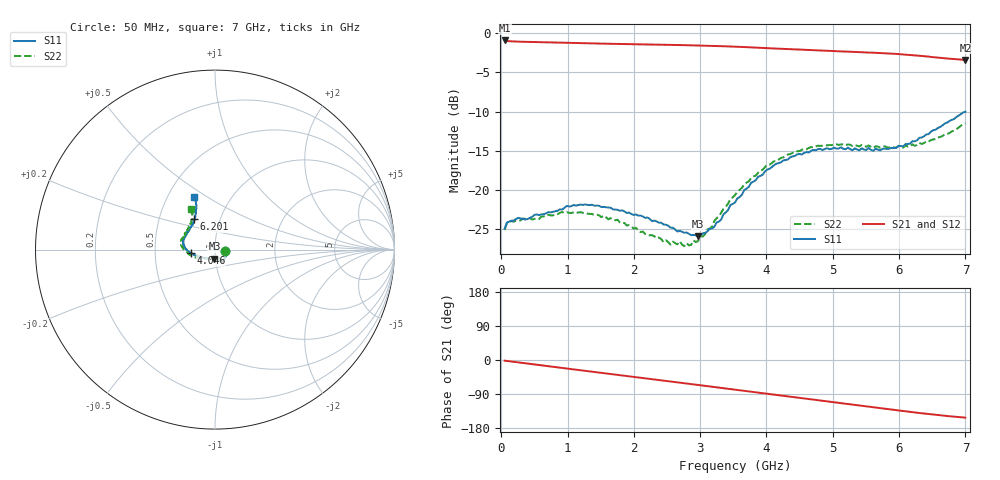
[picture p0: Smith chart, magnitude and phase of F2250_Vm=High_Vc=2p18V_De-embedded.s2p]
! Integrated Device Technology
! Corporate Headquarters
! 6024 Silver Creek Valley Road
! San Jose, CA 95138  USA
! Phone:  1-408-284-8200
! Toll Free:  1-800-223-1366
! Webpage:  http://www.idt.com/
! Timing and RF Division
! 515 Groton Road, Suite 102
! Westford, MA 01886-6024
! Device:  F2250
! Description: Voltage Variable RF Attenuator
! Frequency:  50.0 -  6000.00 MHz
! Package:  3x3 mm Thin QFN Plastic Package: 16 pin
! Ports:  2 RF, 3 DC
!  Pin  1  = GND
!  Pin  2  = NC
!  Pin  3  = RF1  = Port 1
!  Pin  4  = NC
!  Pin  5  = GND
!  Pin  6  = GND
!  Pin  7  = GND
!  Pin  8  = GND
!  Pin  9  = NC
!  Pin 10  = RF2  = Port 2
!  Pin 11  = NC
!  Pin 12  = GND
!  Pin 13  = GND
!  Pin 14  = VCNTRL
!  Pin 15  = VDD
!  Pin 16  = VMODE
! Vcntrl:  2.180 Volts
! Vmode:  +3.300 Volts
! Vdd:  +3.30  Volts
! Current:  1.316 mA
! Data:  The device was measured on a the F2250 evaluation board which has
!  individual transmission lines to the RF pins.  Data was collected
!  using a calibrated network analyzer.  The evaluation board was
!  de-embedded using a TRL calibration technique.
!  The reference plane is the edge of the package pin.
! Misc:  SN 10
!  Action Tracker AT0258
! Date Measured:  2014-11-26
! Date:  2015-10-15  MJV
! Note:
!  Integrated Device Technology supplies this data as a sample of measured
!  data at the package pin for this product.  Your particular data for this
!  product may vary.
!  Data was taken at 25 degrees C.
!  Integrated Device Technology reserves the right to change this data at anytime.
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# GHz S dB R 50
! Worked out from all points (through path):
!   201 points, 50 MHz to 7 GHz, reference 50 ohm
!   highest |S21| = -0.94 dB at 50 MHz (marker M1); lowest = -3.4 dB at 7 GHz (marker M2)
!   group delay of S21, straight-line fit = 61.1 ps
!   lowest |S11| = -25.9 dB at 2.969 GHz (marker M3), VSWR 1.11, Z = 49.4 - j5.01 ohm
!   |S11| at or under -10 dB: start of sweep to end of sweep
!   |S22| runs from -27.2 to -11.5 dB; largest |S21 - S12| = 0.0019
!   S11 on the Smith chart (normalised r, x): 50 MHz: 1.12, -0.02; 4.046 GHz: 0.76, -0.03; 6.201 GHz: 0.75, +0.26; 7 GHz: 0.68, +0.44
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0.05  -24.94 -9.8  -0.94 -1.8  -0.93 -1.8  -25.11 -10.2
0.1195  -24.03 -9.5  -1.03 -3.3  -1.03 -3.2  -24.01 -8.5
0.91875  -22.50 -47.8  -1.22 -21.0  -1.22 -21.1  -22.80 -49.6
1.2315  -21.90 -55.6  -1.29 -27.9  -1.29 -27.9  -22.91 -60.1
1.75275  -22.52 -62.5  -1.38 -39.1  -1.38 -39.1  -23.78 -67.0
2.37825  -24.18 -62.5  -1.47 -52.8  -1.47 -52.8  -26.07 -67.9
2.552  -24.80 -67.1  -1.49 -56.6  -1.49 -56.7  -26.97 -74.5
2.691  -25.22 -74.6  -1.52 -59.7  -1.52 -59.8  -26.54 -81.8
2.7605  -25.45 -76.7  -1.53 -61.3  -1.53 -61.3  -27.16 -86.2
2.969  -25.91 -93.5  -1.57 -66.0  -1.57 -66.0  -26.49 -104.7
3.21225  -24.69 -123.2  -1.63 -71.4  -1.63 -71.5  -23.97 -129.1
3.4555  -21.92 -145.0  -1.70 -76.9  -1.70 -77.0  -21.18 -144.4
3.525  -21.60 -149.4  -1.73 -78.5  -1.73 -78.5  -20.66 -147.7
3.76825  -19.08 -162.4  -1.82 -84.0  -1.82 -84.0  -18.48 -158.8
4.04625  -17.29 -172.1  -1.93 -90.2  -1.93 -90.2  -16.78 -169.3
4.4285  -15.66 177.5  -2.07 -98.6  -2.08 -98.6  -15.07 179.2
4.7065  -14.88 170.5  -2.17 -104.8  -2.18 -104.8  -14.57 173.4
5.054  -14.73 162.2  -2.30 -112.4  -2.30 -112.5  -14.17 166.3
5.85325  -14.73 136.2  -2.60 -130.0  -2.60 -130.1  -14.58 147.5
6.20075  -13.78 124.5  -2.81 -137.7  -2.81 -137.8  -14.18 138.4
6.54825  -12.32 116.3  -3.08 -144.7  -3.08 -144.8  -13.52 127.0
7  -10.02 111.4  -3.41 -152.1  -3.42 -152.2  -11.50 120.8
